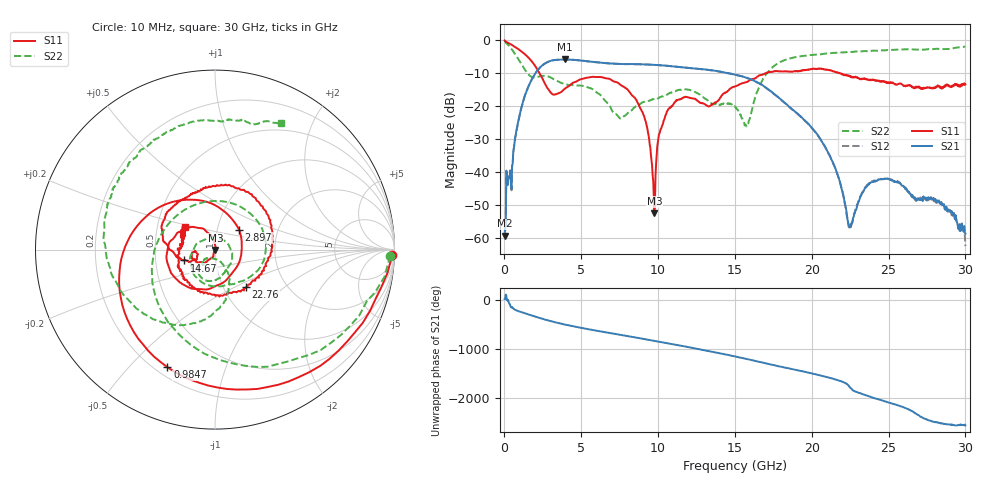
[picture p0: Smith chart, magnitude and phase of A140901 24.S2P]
!  2-Port S-parameters saved by WinCal
! VAR MeasName=S-Parameters (CALIBRATED_DATA) read from VNA (N5244A)
! VAR MeasDate=11/3/2014 9:28:47 AM
! VAR NAME=A140901 24
! VAR FILENAME=A140901 24.S2P
! VAR DATE=11/3/2014 9:28:47 AM
! VAR PHYS_PORTS=1,2
# Hz S RI R 50
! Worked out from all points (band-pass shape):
!   801 points, 10 MHz to 30 GHz, reference 50 ohm
!   highest |S21| = -5.89 dB at 3.909 GHz (marker M1); lowest = -59.4 dB at 10 MHz (marker M2)
!   |S21| within 3 dB of the highest: 2.207 GHz to 12.97 GHz (10.76 GHz wide, 142 % of centre)
!   lowest |S11| = -52.6 dB at 9.757 GHz (marker M3), VSWR 1.00, Z = 50.2 - j0.139 ohm
!   |S11| at or under -10 dB: 2.274 GHz to 17.03 GHz (14.76 GHz wide, 153 % of centre); 21.77172 GHz to 21.81894 GHz (47.21 MHz wide, 0.217 % of centre); 21.83 GHz to end of sweep
!   |S22| runs from -26.2 to -0.2 dB; largest |S21 - S12| = 0.0032
!   S11 on the Smith chart (normalised r, x): 10 MHz: 24, -57; 984.7 MHz: 0.25, -0.65; 2.897 GHz: 1.27, +0.29; 14.67 GHz: 0.70, -0.09; 22.76 GHz: 1.27, -0.58; 30 GHz: 0.69, +0.18
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1e7  0.987 -0.0292  0.000975 0.00044  -0.00142 -0.000412  0.9761 -0.0337
4.5985e8  0.4707 -0.7087  -0.00472 -0.0028  -0.00455 -0.00258  0.3564 -0.636
9.84675e8  -0.2649 -0.6556  -0.0428 0.0573  -0.0427 0.0573  -0.2612 -0.4049
1.884375e9  -0.4128 0.1561  0.2339 0.1542  0.2337 0.1541  -0.0612 0.2644
2.896538e9  0.1337 0.1105  0.2298 -0.4158  0.23 -0.4153  0.272 -0.0616
3.9087e9  0.0626 -0.1697  -0.3813 -0.3351  -0.3811 -0.3352  0.104 -0.1923
5.033325e9  -0.1473 -0.2105  -0.4174 0.2528  -0.4168 0.2531  -0.0345 -0.1999
6.382875e9  -0.27 -0.0312  0.1436 0.4273  0.1433 0.4273  -0.1319 -0.027
8.519662e9  -0.0612 0.1139  0.305 -0.3042  0.3055 -0.3038  0.096 -0.0177
9.231925e9  -0.00697 0.0523  0.0376 -0.4246  0.0376 -0.4247  0.0856 -0.0813
9.75675e9  0.00188 -0.00139  -0.1767 -0.3814  -0.1758 -0.3811  0.0685 -0.1073
1.001916e10  -0.00958 -0.0301  -0.2681 -0.3202  -0.2678 -0.3195  0.057 -0.1172
1.073142e10  -0.0562 -0.0729  -0.3993 -0.063  -0.3991 -0.0624  0.0336 -0.1517
1.234339e10  -0.1275 -0.0173  -0.0335 0.3696  -0.0332 0.3693  -0.0881 -0.14
1.466761e10  -0.1709 -0.0602  0.1956 -0.2413  0.1956 -0.2411  -0.0725 -0.0821
1.5005e10  -0.1907 -0.0512  0.0856 -0.2859  0.0835 -0.286  -0.069 -0.0675
1.579224e10  -0.2311 -0.0151  -0.1644 -0.209  -0.1647 -0.2077  -0.0037 -0.0521
1.729174e10  -0.2935 0.148  -0.0926 0.1431  -0.0909 0.1425  -0.00923 -0.3552
2.002832e10  0.0584 0.3621  0.0202 -0.0409  0.0208 -0.0407  -0.5836 -0.1068
2.276491e10  0.1735 -0.2094  0.000952 -0.00207  0.001 -0.00211  -0.535 0.402
2.501416e10  -0.1903 -0.1118  0.00372 0.00677  0.00379 0.00686  -0.2735 0.6529
3e10  -0.1699 0.1262  0.000752 -0.000869  0.000638 -0.000378  0.3682 0.7037
